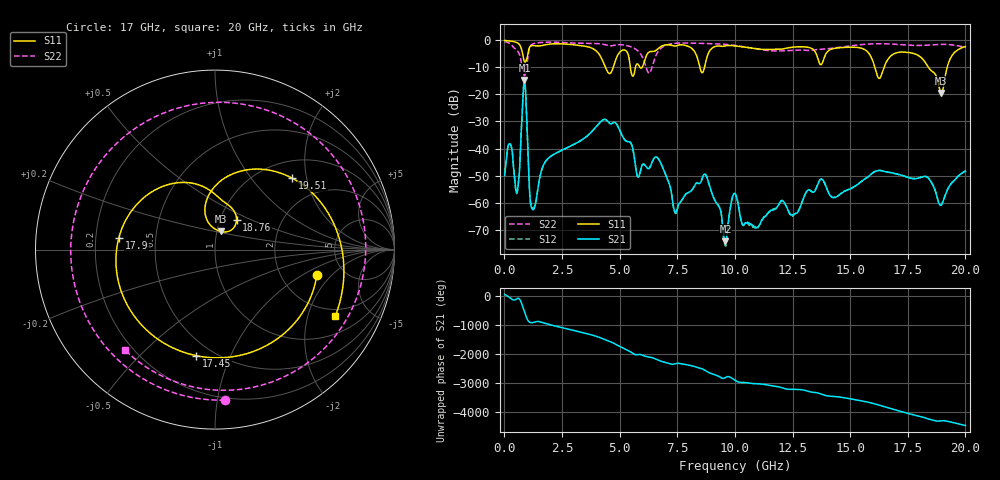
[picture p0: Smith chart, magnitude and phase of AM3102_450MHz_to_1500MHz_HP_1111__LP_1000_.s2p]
!Agilent Technologies,E8364B,MY43040894,A.07.50.67
!Agilent E8364B: A.07.50.67
!Date: Thursday, January 11, 2018 06:50:38
!Correction: S11(Full 2 Port(1,2))
!S21(Full 2 Port(1,2))
!S12(Full 2 Port(1,2))
!S22(Full 2 Port(1,2))
!S2P File: Measurements: S11, S21, S12, S22:
# Hz S  dB  R 50
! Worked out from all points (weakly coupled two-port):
!   1601 points, 10 MHz to 20 GHz, reference 50 ohm
!   highest |S21| = -14.65 dB at 872.1 MHz (marker M1); lowest = -74.3 dB at 9.593 GHz (marker M2)
!   lowest |S11| = -19.5 dB at 18.95 GHz (marker M3), VSWR 1.24, Z = 52.1 + j10.7 ohm
!   |S11| at or under -10 dB: 4.383 GHz to 4.723 GHz (339.6 MHz wide, 7.46 % of centre); 16.07 GHz to 16.47 GHz (397.4 MHz wide, 2.44 % of centre); 18.39 GHz to 19.21 GHz (814.3 MHz wide, 4.33 % of centre)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
!   |S22| runs from -13.1 to -0.4 dB; largest |S21 - S12| = 0.0015
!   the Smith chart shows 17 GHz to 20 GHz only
!   S11 on the Smith chart (normalised r, x): 17 GHz: 3.18, -1.37; 17.45 GHz: 0.41, -0.75; 17.9 GHz: 0.30, +0.06; 18.76 GHz: 1.20, +0.41; 19.51 GHz: 1.36, +1.65; 20 GHz: 1.68, -3.02
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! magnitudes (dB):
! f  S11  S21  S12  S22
! 10 MHz  -0.1  -50.0  -49.4  -0.4
! 247.4 MHz  -0.3  -38.3  -38.4  -1.2
! 572.2 MHz  -1.0  -55.4  -55.6  -3.9
! 872.1 MHz  -7.9  -14.6  -14.7  -13.1
! 1.234 GHz  -2.0  -62.6  -62.1  -1.4
! 1.809 GHz  -1.6  -44.5  -44.5  -0.7
! 3.346 GHz  -2.0  -36.9  -36.9  -1.1
! 6.682 GHz  -3.0  -43.8  -43.8  -4.0
! 7.419 GHz  -2.1  -63.5  -64.0  -1.1
! 8.731 GHz  -8.2  -49.7  -49.7  -1.2
! 9.593 GHz  -2.1  -74.3  -76.1  -1.5
! 10.01 GHz  -2.1  -56.7  -56.6  -1.9
! 10.93 GHz  -3.2  -69.4  -69.2  -3.2
! 13.34 GHz  -3.1  -56.1  -55.9  -3.7
! 16.68 GHz  -6.6  -48.8  -48.8  -1.3
! 17 GHz  -4.7  -49.4  -49.4  -1.5
! 17.45 GHz  -4.4  -50.6  -50.5  -1.8
! 17.9 GHz  -5.4  -51.0  -51.0  -1.9
! 18.76 GHz  -13.9  -57.7  -57.8  -1.6
! 18.95 GHz  -19.5  -60.9  -60.8  -1.5
! 19.51 GHz  -4.6  -51.9  -51.7  -1.8
! 20 GHz  -2.3  -48.4  -48.3  -2.5
